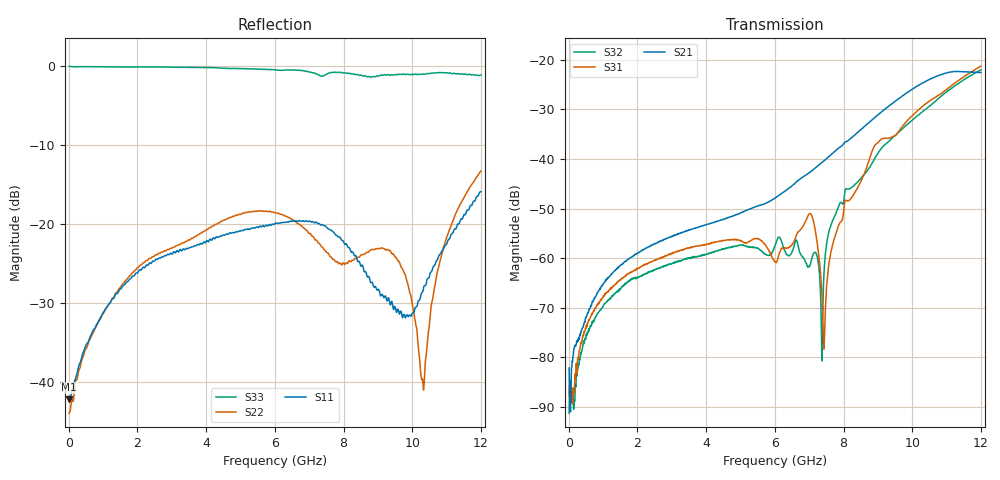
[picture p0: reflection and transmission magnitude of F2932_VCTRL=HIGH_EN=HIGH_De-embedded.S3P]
! Integrated Device Technology
! Corporate Headquarters
! 6024 Silver Creek Valley Road
! San Jose, CA 95138  USA
! Phone:  1-408-284-8200
! Toll Free:  1-800-223-1366
! Webpage:  http://www.idt.com/
! Timing and RF Division
! 515 Groton Road, Suite 102
! Westford, MA 01886-6024
! Device:  F2932
! Description: High Reliability SP2T RF Switch
! Frequency:  0.05 -  8.00 GHz
! Package:  4x4 mm QFN Plastic Package: 16 pin
! Ports:  3 RF, 3 DC
!  Pin  1  = VDD
!  Pin  2  = VCTL
!  Pin  3  = RFC  =  Port 3
!  Pin  4  = GND
!  Pin  5  = EN
!  Pin  6  = GND
!  Pin  7  = GND
!  Pin  8  = GND
!  Pin  9  = RF1  =  Port 1
!  Pin 10  = GND
!  Pin 11  = GND
!  Pin  9  = RF2  =  Port 2
!  Pin 13  = GND
!  Pin 14  = GND
!  Pin 15  = GND
!  Pin 16  = NC
! State:  All Off
! VCTRL:  +2.60 Volts (Logic High)
! EN:  +2.60 Volts (Logic High)
! Voltage:  +5.00 Volts
! Current:  0.417 mA
! Data:  The device was measured on a F2932 evaluation board which has
!  individual transmission lines to the RF pins.  Data was collected
!  using a calibrated network analyzer.  The evaluation board was
!  de-embedded using AFR (Keysight) technique.
!  The reference plane is the edge of the package pin.
! Misc:
!  Action Tracker AT0443
! Date Measured:  2018-10-10
! Date:  2018-10-11  MJV
! Note:
!  Integrated Device Technology supplies this data as a sample of measured
!  data at the package pin for this product.  Your particular data for this
!  product may vary.
!  Data was taken at 25 degrees C.
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# Hz S dB R 50
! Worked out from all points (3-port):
!   1200 points, 10 MHz to 12 GHz, reference 50 ohm
!   strongest paths, dB at 10 MHz, 3.01 GHz, 6.01 GHz, 9.01 GHz, 12 GHz:
!     S21: -82.1, -55.6, -47.8, -31.1, -22.6
!     S31: -87.8, -59.1, -60.7, -36.6, -21.3
!     S32: -91.3, -61.1, -57.3, -38.7, -22.0
!   lowest |S11| = -42.3 dB at 10 MHz (marker M1), VSWR 1.02, Z = 49.2 - j0.00133 ohm
!   |S11| at or under -10 dB: start of sweep to end of sweep
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1e7  -42.26 -179.9  -83.55 3.9  -88.51 40.8
     -82.12 2.1  -44.00 179.0  -87.99 13.4
     -87.80 35.7  -91.25 11.4  -0.07 -0.4
2.21e9  -25.57 50.4  -58.10 87.2  -61.42 74.4
        -58.13 88.0  -24.88 44.4  -63.27 77.4
        -61.31 75.1  -63.24 77.4  -0.17 -43.6
6.01e9  -19.94 -8.4  -47.85 111.6  -60.96 68.6
        -47.85 112.0  -18.60 7.8  -57.34 87.7
        -60.74 69.7  -57.31 87.4  -0.53 -126.2
7.05e9  -19.79 -21.5  -42.51 119.8  -51.07 71.9
        -42.53 120.1  -21.34 -3.4  -60.70 113.3
        -51.09 71.8  -60.75 113.1  -0.84 -147.6
7.44e9  -20.27 -26.1  -40.31 120.6  -77.33 128.2
        -40.31 120.8  -23.34 -16.6  -62.01 -151.7
        -76.66 134.6  -61.96 -151.5  -1.24 -151.4
8.07e9  -22.52 -38.0  -36.52 116.1  -48.32 175.0
        -36.53 116.4  -24.97 -54.5  -46.00 170.8
        -48.30 175.0  -46.01 170.5  -0.94 -164.6
9.58e9  -30.81 -134.9  -27.98 88.7  -34.68 137.9
        -27.99 89.0  -24.69 -105.7  -34.82 138.3
        -34.69 138.1  -34.79 138.3  -1.14 154.4
1.03e10  -28.64 136.6  -24.70 64.2  -29.42 114.2
         -24.70 64.4  -39.65 176.8  -30.53 116.3
         -29.41 114.6  -30.49 116.5  -1.06 137.8
1.092e10  -23.13 107.3  -22.81 38.5  -26.44 91.5
          -22.82 38.9  -22.92 88.5  -26.95 96.7
          -26.41 91.6  -26.91 96.7  -0.91 128.3
1.2e10  -15.95 92.3  -22.58 -0.0  -21.28 48.5
        -22.58 0.4  -13.33 84.4  -22.04 53.6
        -21.30 48.8  -22.04 53.6  -1.20 108.9
